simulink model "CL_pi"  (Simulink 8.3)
settings: Solver=ode23tb  StartTime=0.0  StopTime=6  RelTol=1e-3
InitFcn:
  | ts=100e-6;
StartFcn:
  | close all
undefined symbols (not defined in the file): A, fc, J, Lm, Lr, Ls, P, Rr, Rs, Vdc
libraries: powerlib_extras x1, simulink x1

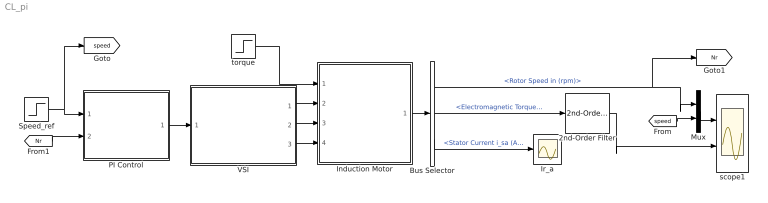
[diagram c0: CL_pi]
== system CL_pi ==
  2nd-Order Filter : powerlib_extras/Control  Blocks/2nd-Order Filter  FilterType=Lowpass  Fo=120  Zeta=0.707  Initialize=off  Vac_Init=[1 45 60]  Vdc_Init=-0.5  PlotResponse=off  param1=[1 500 1]
  Bus Selector : BusSelector  OutputSignals=Mechanical.Rotor Speed in (rpm),Mechanical.Electromagnetic Torque (N*m),Stator Measurement.Stator Current i_sa (A)
  Induction Motor : Subsystem
  Ir_a : Scope
  Mux : Mux  Inputs=2
  PI Control : Subsystem
  Speed_ref : Step  Time=4  Before=1440  After=1200  SampleTime=0
  VSI : Subsystem
  scope1 : Scope  NumInputPorts=2
  torque : Step  Time=2  After=0.5  SampleTime=0
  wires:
  torque/1 -> Induction Motor/1(Torque)
  VSI/1(Va) -> Induction Motor/2(Va)
  VSI/2(Vb) -> Induction Motor/3(Vb)
  VSI/3(Vc) -> Induction Motor/4(Vc)
  Speed_ref/1 -> PI Control/1(speed_ref), [speed]
  PI Control/1(F*) -> VSI/1(F)
  [Nr] -> PI Control/2(Motor_speed)
  Bus Selector/2 -> 2nd-Order Filter/1  "<Electromagnetic Torque (N*m)>"
  Induction Motor/1(m) -> Bus Selector/1
  Bus Selector/1 -> Mux/1, [Nr]  "<Rotor Speed in (rpm)>"
  Bus Selector/3 -> Ir_a/1  "<Stator Current i_sa (A)>"
  Mux/1 -> scope1/1
  [speed] -> Mux/2
  2nd-Order Filter/1 -> scope1/2

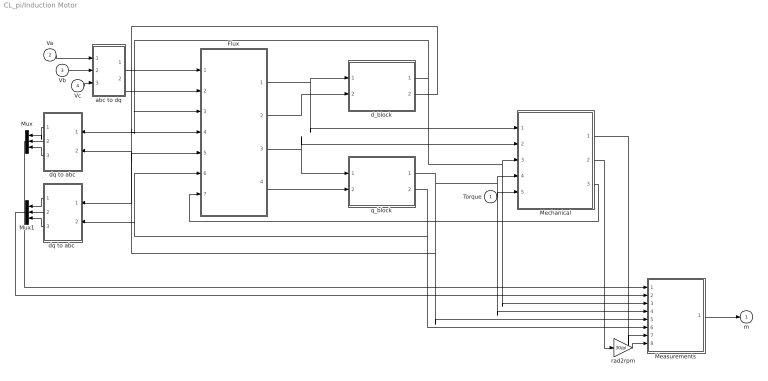
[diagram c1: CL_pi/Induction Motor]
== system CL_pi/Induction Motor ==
  Torque : Inport
  Va : Inport  Port=2
  Vb : Inport  Port=3
  Vc : Inport  Port=4
  Flux : Subsystem
  Measurements : Subsystem
  Mechanical : Subsystem
  Mux : Mux  Inputs=3
  Mux1 : Mux  Inputs=3
  abc to dq : Subsystem
  d_block : Subsystem
  dq to abc : Subsystem
  "dq to abc " : Subsystem
  q_block : Subsystem
  rad2rpm : Gain  Gain=30/pi
  m : Outport
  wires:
  Mechanical/2(omegaR) -> rad2rpm/1
  Mechanical/3(we) -> Flux/7(we)
  Flux/1(shi_ds) -> d_block/1(shi_ds), Mechanical/1(shi_ds)
  Flux/4("shi_qr ") -> q_block/2(shi_qr)
  d_block/1(i_ds) -> Mechanical/3(i_ds), Measurements/3(I_ds), dq to abc/1(I_d), Flux/3(I_ds)
  d_block/2(i_dr) -> Flux/4(I_dr), "dq to abc "/1(I_d)
  q_block/2(i_qr) -> Measurements/6(I_qr), "dq to abc "/2(I_q), Flux/6(I_qr)
  q_block/1(i_qs) -> Mechanical/4(i_qs), Measurements/4(I_dr), Measurements/5(I_qs), dq to abc/2(I_q), Flux/5(I_qs)
  Mechanical/1(Te) -> Measurements/7(Te)
  Torque/1 -> Mechanical/5(tau)
  Flux/2("shi_dr ") -> d_block/2(shi_dr)
  Flux/3(shi_qs) -> q_block/1(shi_qs), Mechanical/2(shi_qs)
  abc to dq/1(V_ds) -> Flux/1(V_ds)
  abc to dq/2(V_qs) -> Flux/2(V_qs)
  Vc/1 -> abc to dq/3(Vc)
  Vb/1 -> abc to dq/2(Vb)
  Va/1 -> abc to dq/1(Va)
  dq to abc/1(i_sa) -> Mux/1
  "dq to abc "/1(i_ra) -> Mux1/1
  dq to abc/2(i_sb) -> Mux/2
  dq to abc/3(i_sc) -> Mux/3
  "dq to abc "/3(i_rc) -> Mux1/3
  "dq to abc "/2(i_rb) -> Mux1/2
  Mux/1 -> Measurements/1(I_s)
  Mux1/1 -> Measurements/2(I_r)
  rad2rpm/1 -> Measurements/8(N)
  Measurements/1(m) -> m/1

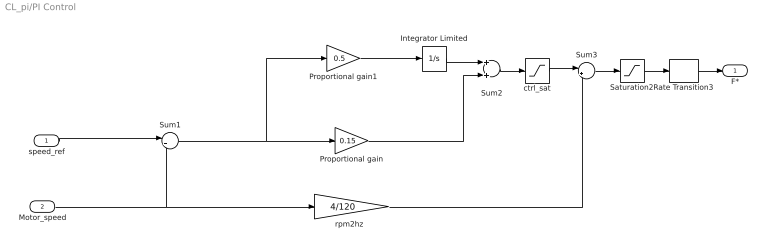
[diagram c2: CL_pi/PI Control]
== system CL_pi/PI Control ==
  speed_ref : Inport
  Motor_speed : Inport  Port=2
  Integrator Limited : Integrator  LimitOutput=on  UpperSaturationLimit=3  LowerSaturationLimit=-3
  Proportional gain : Gain  Gain=0.15
  Proportional gain1 : Gain  Gain=0.5
  Rate Transition3 : RateTransition  OutPortSampleTimeOpt=Inherit
  Saturation2 : Saturate  UpperLimit=120  LowerLimit=0.02
  Sum1 : Sum  Inputs=|+-
  Sum2 : Sum
  Sum3 : Sum  Inputs=|++
  ctrl_sat : Saturate  UpperLimit=30  LowerLimit=-30
  "rpm2hz  " : Gain  Gain=4/120
  F* : Outport
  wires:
  Integrator Limited/1 -> Sum2/1
  Motor_speed/1 -> Sum1/2, "rpm2hz  "/1
  Rate Transition3/1 -> F*/1
  speed_ref/1 -> Sum1/1
  Sum1/1 -> Proportional gain1/1, Proportional gain/1
  Saturation2/1 -> Rate Transition3/1
  Proportional gain/1 -> Sum2/2
  ctrl_sat/1 -> Sum3/1
  Sum3/1 -> Saturation2/1
  Sum2/1 -> ctrl_sat/1
  "rpm2hz  "/1 -> Sum3/2
  Proportional gain1/1 -> Integrator Limited/1

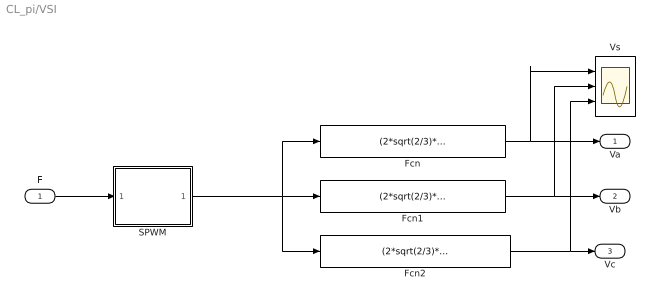
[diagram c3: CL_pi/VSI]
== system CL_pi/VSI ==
  F : Inport
  Fcn : Fcn  Expr=(2*sqrt(2/3)*Vdc/3)*(2*u(1)-u(2)-u(3))
  Fcn1 : Fcn  Expr=(2*sqrt(2/3)*Vdc/3)*(2*u(2)-u(3)-u(1))
  Fcn2 : Fcn  Expr=(2*sqrt(2/3)*Vdc/3)*(2*u(3)-u(2)-u(1))
  SPWM : Subsystem
  Vs : Scope  NumInputPorts=3
  Va : Outport
  Vb : Outport  Port=2
  Vc : Outport  Port=3
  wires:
  SPWM/1(g) -> Fcn2/1, Fcn/1, Fcn1/1
  Fcn1/1 -> Vb/1, Vs/2
  Fcn2/1 -> Vc/1, Vs/3
  Fcn/1 -> Va/1, Vs/1
  F/1 -> SPWM/1(Freq)

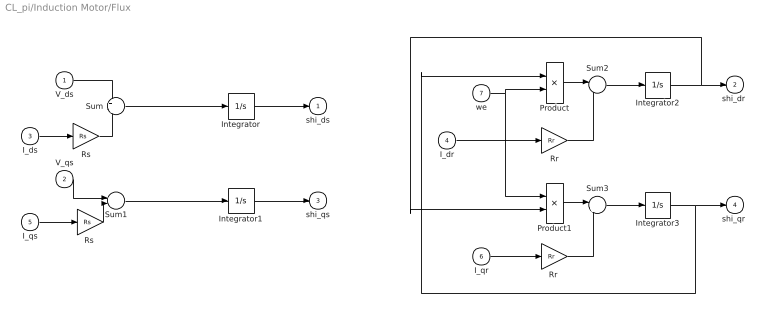
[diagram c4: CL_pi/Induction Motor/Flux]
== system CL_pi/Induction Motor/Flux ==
  V_ds : Inport
  V_qs : Inport  Port=2
  I_ds : Inport  Port=3
  I_dr : Inport  Port=4
  I_qs : Inport  Port=5
  I_qr : Inport  Port=6
  we : Inport  Port=7
  Integrator{,1..3} (4 alike) : Integrator
  Product : Product
  Product1 : Product
  Rr : Gain  Gain=Rr
  "Rr " : Gain  Gain=Rr
  Rs : Gain  Gain=Rs
  "Rs " : Gain  Gain=Rs
  Sum : Sum  Inputs=+|-
  Sum1 : Sum  Inputs=+|-
  Sum2 : Sum  Inputs=|--
  Sum3 : Sum  Inputs=|+-
  shi_ds : Outport
  "shi_dr " : Outport  Port=2
  shi_qs : Outport  Port=3
  "shi_qr " : Outport  Port=4
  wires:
  Sum3/1 -> Integrator3/1
  "Rr "/1 -> Sum3/2
  Product1/1 -> Sum3/1
  I_qr/1 -> "Rr "/1
  Integrator2/1 -> "shi_dr "/1, Product1/2
  Sum2/1 -> Integrator2/1
  Product/1 -> Sum2/1
  Rr/1 -> Sum2/2
  I_dr/1 -> Rr/1
  Integrator3/1 -> "shi_qr "/1, Product/1
  we/1 -> Product1/1, Product/2
  "Rs "/1 -> Sum1/2
  Rs/1 -> Sum/2
  Integrator1/1 -> shi_qs/1
  Integrator/1 -> shi_ds/1
  Sum1/1 -> Integrator1/1
  V_qs/1 -> Sum1/1
  I_qs/1 -> "Rs "/1
  Sum/1 -> Integrator/1
  V_ds/1 -> Sum/1
  I_ds/1 -> Rs/1

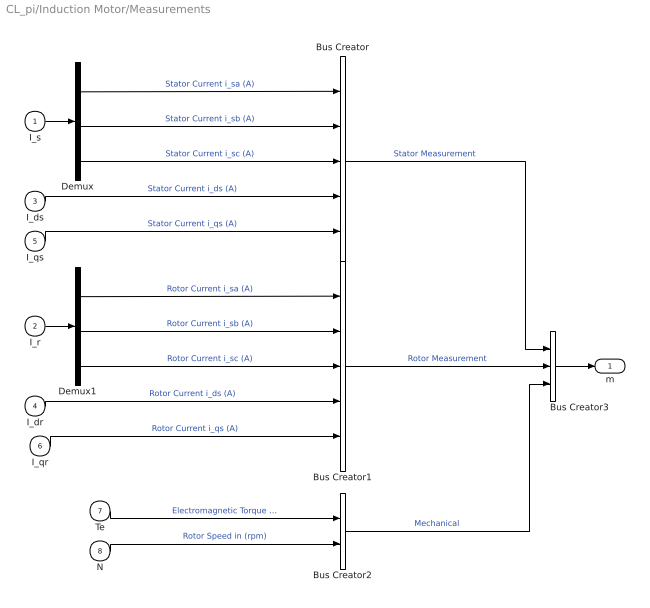
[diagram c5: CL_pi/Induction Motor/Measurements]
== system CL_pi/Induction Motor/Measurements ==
  I_s : Inport
  I_r : Inport  Port=2
  I_ds : Inport  Port=3
  I_dr : Inport  Port=4
  I_qs : Inport  Port=5
  I_qr : Inport  Port=6
  Te : Inport  Port=7
  N : Inport  Port=8
  Bus Creator : BusCreator  Inputs=5
  Bus Creator1 : BusCreator  Inputs=5
  Bus Creator2 : BusCreator  Inputs=2
  Bus Creator3 : BusCreator  Inputs=3
  Demux : Demux  Outputs=3
  Demux1 : Demux  Outputs=3
  m : Outport
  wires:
  Bus Creator3/1 -> m/1
  Bus Creator2/1 -> Bus Creator3/3  "Mechanical"
  Bus Creator1/1 -> Bus Creator3/2  "Rotor Measurement"
  Bus Creator/1 -> Bus Creator3/1  "Stator Measurement"
  N/1 -> Bus Creator2/2  "Rotor Speed in (rpm)"
  Te/1 -> Bus Creator2/1  "Electromagnetic Torque (N*m)"
  I_qr/1 -> Bus Creator1/5  "Rotor Current i_qs (A)"
  I_dr/1 -> Bus Creator1/4  "Rotor Current i_ds (A)"
  Demux1/3 -> Bus Creator1/3  "Rotor Current i_sc (A)"
  Demux1/2 -> Bus Creator1/2  "Rotor Current i_sb (A)"
  Demux1/1 -> Bus Creator1/1  "Rotor Current i_sa (A)"
  I_r/1 -> Demux1/1
  I_qs/1 -> Bus Creator/5  "Stator Current i_qs (A)"
  I_ds/1 -> Bus Creator/4  "Stator Current i_ds (A)"
  Demux/3 -> Bus Creator/3  "Stator Current i_sc (A)"
  Demux/2 -> Bus Creator/2  "Stator Current i_sb (A)"
  Demux/1 -> Bus Creator/1  "Stator Current i_sa (A)"
  I_s/1 -> Demux/1

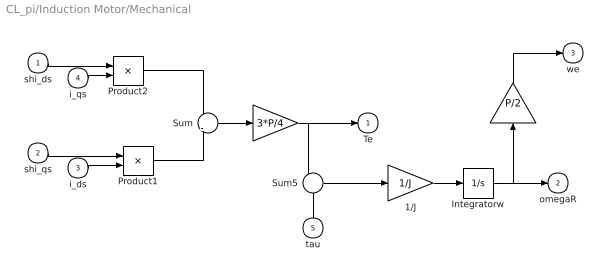
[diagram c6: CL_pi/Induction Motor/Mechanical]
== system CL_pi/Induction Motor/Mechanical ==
  shi_ds : Inport
  shi_qs : Inport  Port=2
  i_ds : Inport  Port=3
  i_qs : Inport  Port=4
  tau : Inport  Port=5
  " " : Gain  Gain=P/2
  "  " : Gain  Gain=3*P/4
  1/J : Gain  Gain=1/J
  Integratorw : Integrator
  Product1 : Product
  Product2 : Product
  Sum : Sum  Inputs=+|-
  Sum5 : Sum  Inputs=+-
  Te : Outport
  omegaR : Outport  Port=2
  we : Outport  Port=3
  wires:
  " "/1 -> we/1
  Integratorw/1 -> omegaR/1, " "/1
  1/J/1 -> Integratorw/1
  Sum5/1 -> 1/J/1
  tau/1 -> Sum5/2
  "  "/1 -> Sum5/1, Te/1
  Sum/1 -> "  "/1
  Product2/1 -> Sum/1
  Product1/1 -> Sum/2
  i_ds/1 -> Product1/2
  shi_qs/1 -> Product1/1
  i_qs/1 -> Product2/2
  shi_ds/1 -> Product2/1

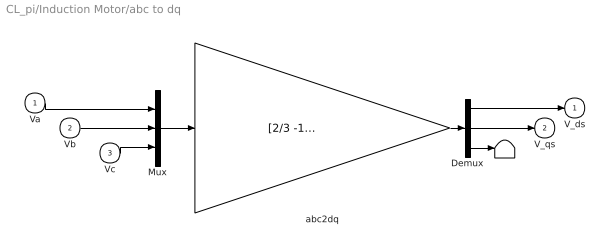
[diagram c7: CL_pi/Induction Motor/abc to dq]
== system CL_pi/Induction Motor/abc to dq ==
  Va : Inport
  Vb : Inport  Port=2
  Vc : Inport  Port=3
  "            " : Terminator
  Demux : Demux  Outputs=3
  Mux : Mux  Inputs=3
  abc2dq : Gain  Gain=[2/3 -1/3 -1/3; 0 sqrt(3)/3 -sqrt(3)/3; 1/3 1/3 1/3]  Multiplication=Matrix(K*u)
  V_ds : Outport
  V_qs : Outport  Port=2
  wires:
  Mux/1 -> abc2dq/1
  abc2dq/1 -> Demux/1
  Demux/2 -> V_qs/1
  Demux/1 -> V_ds/1
  Va/1 -> Mux/1
  Vb/1 -> Mux/2
  Vc/1 -> Mux/3
  Demux/3 -> "            "/1

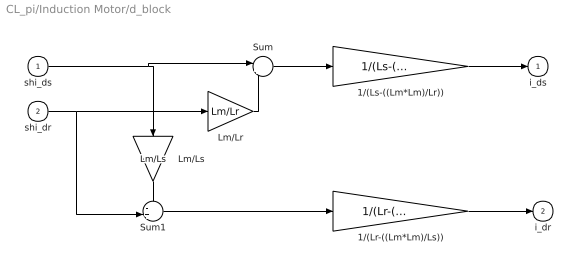
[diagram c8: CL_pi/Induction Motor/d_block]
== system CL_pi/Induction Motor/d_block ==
  shi_ds : Inport
  shi_dr : Inport  Port=2
  1/(Lr-((Lm*Lm)/Ls)) : Gain  Gain=1/(Lr-((Lm*Lm)/Ls))
  1/(Ls-((Lm*Lm)/Lr)) : Gain  Gain=1/(Ls-((Lm*Lm)/Lr))
  Lm/Lr : Gain  Gain=Lm/Lr
  Lm/Ls : Gain  Gain=Lm/Ls
  Sum : Sum  Inputs=|+-
  Sum1 : Sum  Inputs=-+|
  i_ds : Outport
  i_dr : Outport  Port=2
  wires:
  Sum1/1 -> 1/(Lr-((Lm*Lm)/Ls))/1
  Lm/Ls/1 -> Sum1/1
  Sum/1 -> 1/(Ls-((Lm*Lm)/Lr))/1
  Lm/Lr/1 -> Sum/2
  shi_dr/1 -> Sum1/2, Lm/Lr/1
  shi_ds/1 -> Lm/Ls/1, Sum/1
  1/(Lr-((Lm*Lm)/Ls))/1 -> i_dr/1
  1/(Ls-((Lm*Lm)/Lr))/1 -> i_ds/1

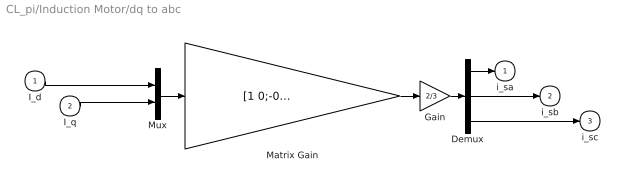
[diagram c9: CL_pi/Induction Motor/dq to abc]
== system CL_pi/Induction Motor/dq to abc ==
  I_d : Inport
  I_q : Inport  Port=2
  Demux : Demux  Outputs=3
  Gain : Gain  Gain=2/3
  Matrix Gain : Gain  Gain=[1 0;-0.5 -sqrt(3)/2;-0.5 sqrt(3)/2]  Multiplication=Matrix(K*u)
  Mux : Mux  Inputs=2
  i_sa : Outport
  i_sb : Outport  Port=2
  i_sc : Outport  Port=3
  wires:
  Demux/1 -> i_sa/1
  Demux/3 -> i_sc/1
  I_q/1 -> Mux/2
  I_d/1 -> Mux/1
  Demux/2 -> i_sb/1
  Matrix Gain/1 -> Gain/1
  Gain/1 -> Demux/1
  Mux/1 -> Matrix Gain/1

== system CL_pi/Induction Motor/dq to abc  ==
  I_d : Inport
  I_q : Inport  Port=2
  Demux : Demux  Outputs=3
  Gain : Gain  Gain=2/3
  Matrix Gain : Gain  Gain=[1 0;-0.5 -sqrt(3)/2;-0.5 sqrt(3)/2]  Multiplication=Matrix(K*u)
  Mux : Mux  Inputs=2
  i_ra : Outport
  i_rb : Outport  Port=2
  i_rc : Outport  Port=3
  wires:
  Mux/1 -> Matrix Gain/1
  Gain/1 -> Demux/1
  Matrix Gain/1 -> Gain/1
  Demux/2 -> i_rb/1
  I_d/1 -> Mux/1
  I_q/1 -> Mux/2
  Demux/3 -> i_rc/1
  Demux/1 -> i_ra/1

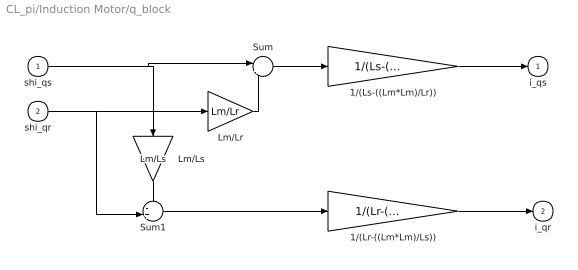
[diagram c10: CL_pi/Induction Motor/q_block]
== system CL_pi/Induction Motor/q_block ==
  shi_qs : Inport
  shi_qr : Inport  Port=2
  1/(Lr-((Lm*Lm)/Ls)) : Gain  Gain=1/(Lr-((Lm*Lm)/Ls))
  1/(Ls-((Lm*Lm)/Lr)) : Gain  Gain=1/(Ls-((Lm*Lm)/Lr))
  Lm/Lr : Gain  Gain=Lm/Lr
  Lm/Ls : Gain  Gain=Lm/Ls
  Sum : Sum  Inputs=|+-
  Sum1 : Sum  Inputs=-+|
  i_qs : Outport
  i_qr : Outport  Port=2
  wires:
  Sum1/1 -> 1/(Lr-((Lm*Lm)/Ls))/1
  Lm/Ls/1 -> Sum1/1
  Sum/1 -> 1/(Ls-((Lm*Lm)/Lr))/1
  Lm/Lr/1 -> Sum/2
  shi_qr/1 -> Lm/Lr/1, Sum1/2
  shi_qs/1 -> Lm/Ls/1, Sum/1
  1/(Lr-((Lm*Lm)/Ls))/1 -> i_qr/1
  1/(Ls-((Lm*Lm)/Lr))/1 -> i_qs/1

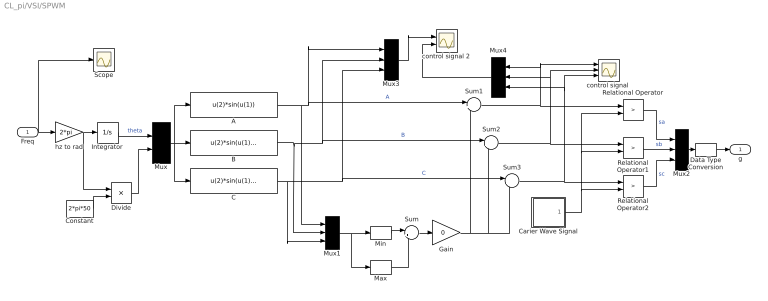
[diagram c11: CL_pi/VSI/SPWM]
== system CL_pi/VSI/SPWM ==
  Freq : Inport
  A : Fcn  Expr=u(2)*sin(u(1))
  B : Fcn  Expr=u(2)*sin(u(1)-2*pi/3)
  C : Fcn  Expr=u(2)*sin(u(1)+2*pi/3)
  Carier Wave Signal : Subsystem
  Constant : Constant  Value=2*pi*50
  Data Type Conversion : DataTypeConversion
  Divide : Product  Inputs=*/
  Gain : Gain  Gain=0
  Integrator : Integrator
  Max : MinMax  Function=max
  Min : MinMax
  Mux : Mux  Inputs=2
  Mux{1..4} (4 alike) : Mux  Inputs=3
  Relational Operator : RelationalOperator  Operator=>  OutDataTypeStr=boolean
  Relational Operator1 : RelationalOperator  Operator=>  OutDataTypeStr=boolean
  Relational Operator2 : RelationalOperator  Operator=>  OutDataTypeStr=boolean
  Scope : Scope
  Sum{,1..3} (4 alike) : Sum  Inputs=|++
  "control signal " : Scope  NumInputPorts=3
  control signal 2 : Scope  NumInputPorts=2
  hz to rad : Gain  Gain=2*pi
  g : Outport
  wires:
  Mux4/1 -> control signal 2/2
  Mux3/1 -> control signal 2/1
  Constant/1 -> Divide/2
  Divide/1 -> Mux/2
  Gain/1 -> Sum1/2, Sum3/2, Sum2/2
  Freq/1 -> hz to rad/1, Scope/1
  C/1 -> Mux3/3, Sum3/1, Mux1/3  "C"
  Mux/1 -> C/1, A/1, B/1
  Integrator/1 -> Mux/1  "theta"
  A/1 -> Mux3/1, Sum1/1, Mux1/1  "A"
  hz to rad/1 -> Divide/1, Integrator/1
  B/1 -> Mux3/2, Sum2/1, Mux1/2  "B"
  Min/1 -> Sum/1
  Max/1 -> Sum/2
  Carier Wave Signal/1("Carier Wave ") -> Relational Operator2/2, Relational Operator1/2, Relational Operator/2
  Relational Operator2/1 -> Mux2/3  "sc"
  Relational Operator1/1 -> Mux2/2  "sb"
  Relational Operator/1 -> Mux2/1  "sa"
  Mux1/1 -> Max/1, Min/1
  Sum/1 -> Gain/1
  Sum1/1 -> Mux4/1, "control signal "/1, Relational Operator/1
  Sum2/1 -> Mux4/2, "control signal "/2, Relational Operator1/1
  Sum3/1 -> Mux4/3, "control signal "/3, Relational Operator2/1
  Mux2/1 -> Data Type Conversion/1
  Data Type Conversion/1 -> g/1

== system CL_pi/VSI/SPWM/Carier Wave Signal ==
  Carier Wave : simulink/Sources/Repeating Sequence  rep_seq_t=[0 0.25 0.5 0.75 1]./fc  rep_seq_y=[0 1 0 -1 0].*A
  "Carier Wave " : Outport
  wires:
  Carier Wave/1 -> "Carier Wave "/1  "0 delay"
